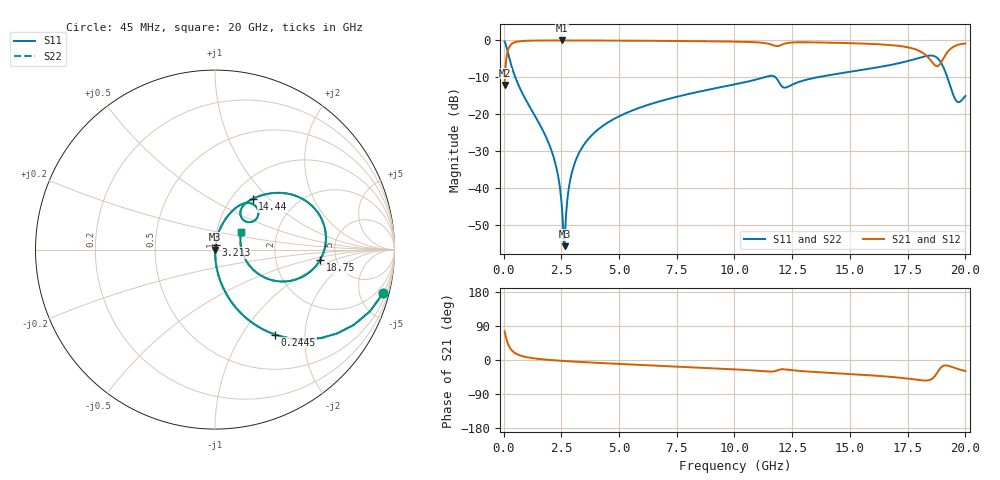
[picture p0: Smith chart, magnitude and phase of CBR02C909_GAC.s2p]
! S-parameter model data by Modelithics Inc.  support@modelithics.com 813-866-6335  Tampa FL USA
! S-Parameter data specifications:
! Substrate: 20-mil Rogers 4350B, substrate thickness, H=0.508mm, Dielectric constant, Er=3.75
! PCB Mounting Pad Footprint: Pad width, PadW=0.32mm , Pad length, PadL=0.37mm , Pad gap, PadG (edge-to-edge)=0.19mm , Reference planes=0.93mm apart
#  GHz  S  MA  R 50
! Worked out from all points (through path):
!   801 points, 45 MHz to 20 GHz, reference 50 ohm
!   highest |S21| = -0.01 dB at 2.539 GHz (marker M1); lowest = -12.1 dB at 45 MHz (marker M2)
!   group delay of S21, straight-line fit = 7.5 ps
!   lowest |S11| = -55.8 dB at 2.639 GHz (marker M3), VSWR 1.00, Z = 50.2 + j0.0534 ohm
!   |S11| at or under -10 dB: 508.4 MHz to 11.29 GHz (10.79 GHz wide, 183 % of centre); 11.77 GHz to 13.6 GHz (1.821 GHz wide, 14.4 % of centre); 19.22 GHz to end of sweep
!   |S22| runs from -55.8 to -0.3 dB; largest |S21 - S12| = 0
!   S11 on the Smith chart (normalised r, x): 45 MHz: 0.99, -7.80; 244.6 MHz: 1.00, -1.42; 3.213 GHz: 1.01, +0.05; 14.44 GHz: 1.24, +0.80; 18.75 GHz: 3.72, -0.68; 20 GHz: 1.31, +0.27
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0.045  0.9688 -14.4  0.2476 75.6  0.2476 75.6  0.9688 -14.4
0.24455  0.5808 -54.7  0.8135 35.3  0.8135 35.3  0.5808 -54.7
0.668594  0.2391 -76.6  0.9701 13.2  0.9701 13.2  0.2391 -76.6
2.090387  0.03098 -87.8  0.9981 -0.3  0.9981 -0.3  0.03098 -87.8
2.364769  0.01424 -85.8  0.9984 -1.6  0.9984 -1.6  0.01424 -85.8
2.539375  0.004809 -74.5  0.9985 -2.3  0.9985 -2.3  0.004809 -74.5
2.63915  0.001613 19.3  0.9985 -2.7  0.9985 -2.7  0.001613 19.3
2.888587  0.01287 79.4  0.9983 -3.6  0.9983 -3.6  0.01287 79.4
3.212856  0.02733 81.8  0.9979 -4.8  0.9979 -4.8  0.02733 81.8
3.387462  0.03465 81.9  0.9977 -5.4  0.9977 -5.4  0.03465 81.9
4.584763  0.07923 79.5  0.9949 -9.2  0.9949 -9.2  0.07923 79.5
6.704981  0.1473 73.9  0.9866 -15.2  0.9866 -15.2  0.1473 73.9
10.0225  0.2537 64.1  0.962 -24.8  0.962 -24.8  0.2537 64.1
11.74362  0.322 41.5  0.8475 -29.5  0.8475 -29.5  0.322 41.5
13.36496  0.3055 56.7  0.9406 -31.2  0.9406 -31.2  0.3055 56.7
14.43754  0.3516 53.5  0.9271 -35.1  0.9271 -35.1  0.3516 53.5
16.68248  0.4594 43.4  0.868 -44.1  0.868 -44.1  0.4594 43.4
18.02944  0.5831 26.5  0.7133 -53.1  0.7133 -53.1  0.5831 26.5
18.75281  0.5874 -5.8  0.4474 -36.1  0.4474 -36.1  0.5874 -5.8
19.10203  0.3949 -26.6  0.6101 -14.4  0.6101 -14.4  0.3949 -26.6
19.6009  0.1522 -4.7  0.8535 -22.3  0.8535 -22.3  0.1522 -4.7
20  0.176 34.2  0.9082 -29.2  0.9082 -29.2  0.176 34.2
